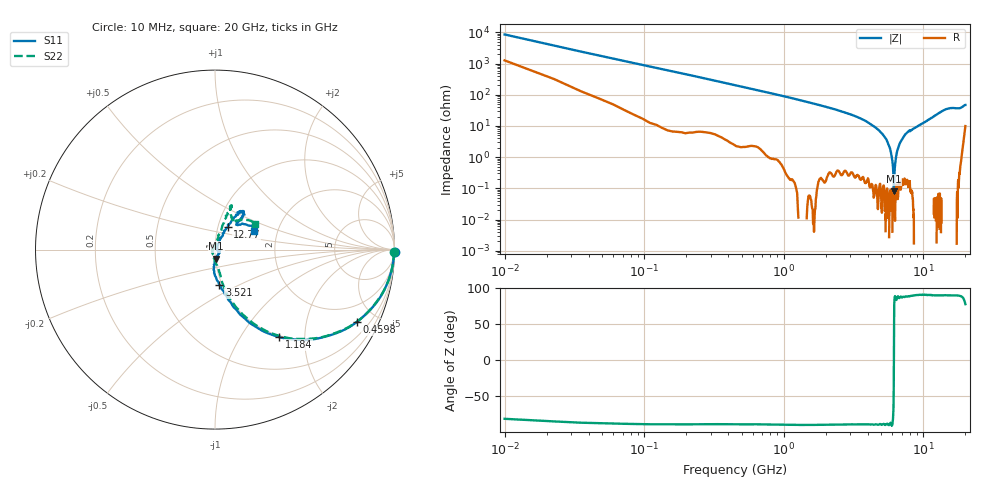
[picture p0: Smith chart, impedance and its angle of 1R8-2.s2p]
!Keysight Technologies,P5008B,MY61100088,A.16.20.02
!Date: Monday, May 27, 2024 14:07:10
!Correction: S11(C  2-Port  )
!S21(C  2-Port  )
!S12(C  2-Port  )
!S22(C  2-Port  )
!S2P File: Measurements: S11, S21, S12, S22:
# Hz S  dB  R 50
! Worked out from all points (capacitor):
!   1601 points, 10 MHz to 20 GHz, reference 50 ohm
!   read as one part in series: C = 1.76 pF near 110 MHz
!   lowest |Z| = 79.5 mohm at 6.144 GHz (marker M1)
!   series resonance near 6.147 GHz, so ESL is about 380 pH
!   S11 on the Smith chart (normalised r, x): 10 MHz: open; 459.8 MHz: 1.03, -3.89; 1.184 GHz: 0.98, -1.49; 3.521 GHz: 0.97, -0.40; 12.77 GHz: 1.11, +0.28; 20 GHz: 1.52, +0.34
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1e7  0.00 -0.7  -38.68 80.9  -38.68 81.0  -0.02 -0.7
1.224438e8  -0.11 -7.9  -17.35 81.3  -17.36 81.3  -0.10 -7.8
1.724188e8  -0.19 -11.0  -14.59 78.4  -14.60 78.4  -0.18 -10.8
4.59775e8  -1.05 -27.1  -6.95 62.4  -6.96 62.4  -1.03 -26.9
1.184412e9  -4.39 -53.8  -1.97 36.5  -1.98 36.5  -4.38 -52.9
1.971519e9  -8.11 -68.5  -0.73 22.0  -0.74 22.0  -8.05 -66.7
3.345831e9  -13.41 -80.8  -0.19 9.8  -0.20 9.8  -13.56 -76.7
3.520744e9  -14.10 -82.9  -0.17 8.8  -0.18 8.8  -14.28 -77.6
6.144431e9  -25.94 -81.9  0.02 -2.9  0.00 -2.9  -25.89 -94.7
6.681662e9  -28.70 -68.4  0.02 -4.6  0.01 -4.6  -29.37 -103.8
7.656175e9  -31.41 -20.1  0.03 -7.4  0.02 -7.4  -36.96 -164.5
8.268369e9  -32.44 -28.7  0.03 -9.1  0.02 -9.1  -37.19 -164.1
8.830588e9  -36.76 -17.0  0.04 -10.6  0.03 -10.6  -41.62 165.9
9.530238e9  -39.84 25.9  0.05 -12.4  0.04 -12.4  -40.22 115.8
1.0005e10  -34.22 53.6  0.05 -13.6  0.04 -13.6  -34.38 90.8
1.10045e10  -25.25 65.6  0.04 -16.2  0.03 -16.2  -25.94 77.6
1.276612e10  -16.87 60.8  -0.03 -20.7  -0.04 -20.7  -16.93 72.7
1.334083e10  -14.87 60.0  -0.08 -22.2  -0.09 -22.2  -14.94 72.1
1.499001e10  -11.77 55.8  -0.22 -26.2  -0.23 -26.2  -11.78 69.4
1.667666e10  -12.30 50.6  -0.19 -29.1  -0.20 -29.1  -12.26 69.0
1.836332e10  -14.81 49.4  -0.13 -33.6  -0.13 -33.7  -14.70 57.1
2e10  -12.25 25.6  -1.03 -38.3  -1.04 -38.4  -11.63 32.5
